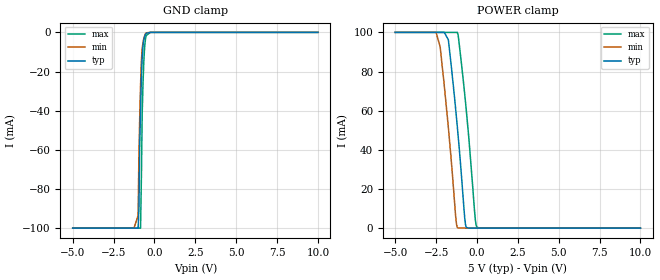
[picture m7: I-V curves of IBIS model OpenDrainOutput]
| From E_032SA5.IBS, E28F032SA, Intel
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|********************Open Drain Output Model************************
[Model]   OpenDrainOutput
Model_type   Open_drain
|   for RY/BY# pin 53
Vinl = 0.8V
Vinh = 2.0V
| Variable   typ   min   max
C_comp   9.61p   NA   11.6p
[Voltage Range]   5.0V   4.5V   5.5V
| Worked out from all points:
|   GND clamp passes 1 mA (typ) near -0.54 V on its own axis
|   POWER clamp passes 1 mA (typ) near -0.67 V on its own axis
[Pulldown]
| [Pullup] and [Pulldown] IV curves include only the current through
| the channels of output driver transistors when outputs are enabled
| with OE# = VIL.  Although the output driver transistors have np and
| pn diodes inherently created by CMOS IC fabrication between the
| drain and bulk of n-channel and p-channel CMOS transistors,
| the current through these junction diodes is not included in
| [Pullup] or [Pulldown].  Instead that drain/bulk diode current is
| included in the [POWER_clamp] or [GND_clamp] sections, which are
| not dependent on the state of OE# or output data value.  The RY/BY#
| Pulldown information is not provided for this device.  The table
| below is for the compatibility with some IBIS parsers.
|Voltage  I(typ)   I(min)   I(max)
-5V       0A         0A         0A
10V       0A         0A         0A
[GND_clamp]
| [POWER_clamp] and [GND_clamp] IV curves describe ESD protection
| circuits PLUS some np and pn diodes which exist between the
| drain and bulk of n-channel and p-channel CMOS transistors.
| These drain/bulk diodes are inherent in CMOS IC fabrication,
| and are visible on the node of the I/O pin at all times.
| Even the drain/bulk diodes of output driver [Pullup] and [Powerdown]
| transistors are included in [POWER_clamp] or [GND_clamp], because
| these diodes contribute to I/O pin current even when the
| chip outputs are tristated by OE# = VIH.
| For example, when V forced on the I/O pin is large, we are
| forward biasing the pn diode at the drain/bulk interface in the
| p-channel pullup transistor.  Similarly, when V forced on the
| I/O pin is sufficiently negative with respect to the substrate
| ground, we are forward biasing the np diode at the drain/bulk
| interface in the n-channel pulldown transistor.  The effects
| of these diodes are included in [POWER_clamp] or [GND_clamp].
|Voltage  I(typ)   I(min)   I(max)
-5V       -99.85mA   -99.86mA   -99.85mA
-1.25V    -99.85mA   -99.86mA   -99.85mA
-1V       -99.85mA   -93.36mA   -99.85mA
-950mV    -90.34mA   -63.24mA   -99.85mA
-900mV    -57.16mA   -42.82mA   -99.85mA
-850mV    -38.91mA   -26.66mA   -99.85mA
-800mV    -23.28mA   -14.71mA   -74.74mA
-750mV    -12.68mA   -8.348mA   -41.38mA
-700mV    -6.759mA   -5.06mA    -26.01mA
-600mV    -2.156mA   -1.643mA   -7.325mA
-500mV    -423.7uA   -221.5uA   -1.566mA
10V       0A         0A         0A
[Pullup]
| (Voltages for [Pullup] and [POWER_clamp] are specified with
| negative respect to Vcc.  Reference the IBIS documentation
| for more information regarding Vtable = Vcc - Voutput.
| This method keeps -Vds constant for the values in all three
| columns across a line of the table.)
| [Pullup] and [Pulldown] IV curves include only the current through
| the channels of output driver transistors when outputs are enabled
| with OE# = VIL.  Although the output driver transistors have np and
| pn diodes inherently created by CMOS IC fabrication between the
| drain and bulk of n-channel and p-channel CMOS transistors,
| the current through these junction diodes is not included in
| [Pullup] or [Pulldown].  Instead that drain/bulk diode current is
| included in the [POWER_clamp] or [GND_clamp] sections, which are
| not dependent on the state of OE# or output data value.
|   Voltage  I(typ)   I(min)   I(max)
-5V       0A         0A         0A
10V       0A         0A         0A
[POWER_clamp]
| (Voltages for [Pullup] and [POWER_clamp] are specified with
| negative respect to Vcc.  Reference the IBIS documentation
| for more information regarding Vtable = Vcc - Voutput.
| This method keeps -Vds constant for the values in all three
| columns across a line of the table.
| [POWER_clamp] and [GND_clamp] IV curves describe ESD protection
| circuits PLUS some np and pn diodes which exist between the
| drain and bulk of n-channel and p-channel CMOS transistors.
| These drain/bulk diodes are inherent in CMOS IC fabrication,
| and are visible on the node of the I/O pin at all times.
| Even the drain/bulk diodes of output driver [Pullup] and [Powerdown]
| transistors are included in [POWER_clamp] or [GND_clamp], because
| these diodes contribute to I/O pin current even when the
| chip outputs are tristated by OE# = VIH.
| For example, when V forced on the I/O pin is large, we are
| forward biasing the pn diode at the drain/bulk interface in the
| p-channel pullup transistor.  Similarly, when V forced on the
| I/O pin is sufficiently negative with respect to the substrate
| ground, we are forward biasing the np diode at the drain/bulk
| interface in the n-channel pulldown transistor.  The effects
| of these diodes are included in [POWER_clamp] or [GND_clamp].
|Voltage  I(typ)   I(min)   I(max)
-5V       100mA      100mA      100mA
-2.5V     100mA      100mA      100mA
-2.25V    100mA      92.59mA    100mA
-1.75V    96.25mA    51.53mA    100mA
-1.3V     60.58mA    5.804mA    100mA
-1.2V     51.74mA    365.3uA    100mA
-1.1V     42.39mA    0A         95.1mA
-700mV    1.826mA    0A         64.4mA
-500mV    1.279uA    0A         46.44mA
-100mV    0A         0A         4.387mA
0V        0A         0A         398.5uA
10V       0A         0A         0A
[Ramp]
| The RY/BY# Ramp information is not provided for this devide.  The table
| below is for the compatibility with some IBIS parsers.
|Variable   typ   min   max
dV/dt_r   0V/0ns   0V/0ns   0V/0ns
dV/dt_f   0V/0ns   0V/0ns   0V/0ns
